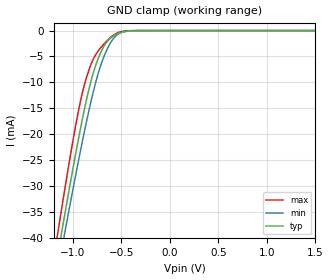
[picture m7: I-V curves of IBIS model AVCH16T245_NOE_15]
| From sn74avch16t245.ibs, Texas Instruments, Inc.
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[Model]   AVCH16T245_NOE_15
Model_type  Input
Vinl=0.49
Vinh=1.04
| variable   typ   min   max
C_comp   2.96pF   2.49pF   3.41pF
[Temperature Range]   40   100   -40
| Ambient temperature   25   85   -40
[Voltage range]   1.5   1.4   1.6
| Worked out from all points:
|   GND clamp passes 1 mA (typ) near -0.58 V on its own axis
[GND Clamp]
| AVCH16T245_NOE_15
|   Voltage   I(typ)   I(min)   I(max)
-4.6V     -463.5mA   -440.8mA   -490.1mA
-1.165V   -44.34mA   -47.36mA   -40.17mA
-1.14V    -41.6mA    -44.78mA   -37.2mA
-1.115V   -38.87mA   -42.22mA   -34.26mA
-1.09V    -36.17mA   -39.68mA   -31.36mA
-1.065V   -33.49mA   -37.15mA   -28.49mA
-945mV    -21.15mA   -25.38mA   -15.71mA
-850mV    -12.51mA   -16.73mA   -8.451mA
-710mV    -4.106mA   -6.531mA   -3.225mA
-630mV    -1.768mA   -2.95mA    -1.612mA
-545mV    -660.8uA   -840.9uA   -480.8uA
1.5V      143.7pA    862pA      25.61pA
